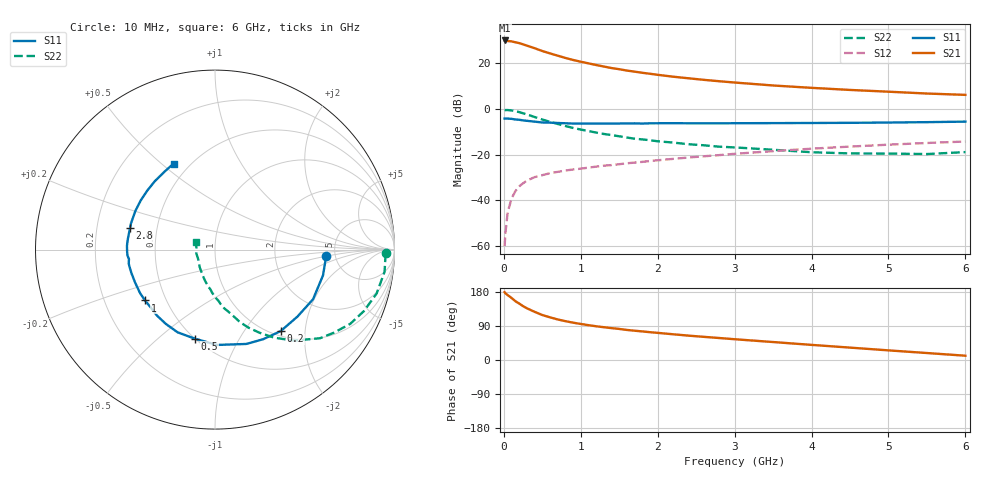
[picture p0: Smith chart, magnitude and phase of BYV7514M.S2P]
! SIEMENS Small Signal Semiconductors
! BFY420
! Si NPN RF SIEGET Grounded Emitter Transistor in MICRO-X
! VCE = 0.75 V  IC = 14 mA
! Common Emitter S-Parameters:  October  1996
# GHz  S  MA  R  50
!  f  S11  S21  S12  S22
! GHz  MAG  ANG  MAG  ANG  MAG  ANG  MAG  ANG
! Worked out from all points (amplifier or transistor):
!   36 points, 10 MHz to 6 GHz, reference 50 ohm
!   highest |S21| = 30.0 dB at 10 MHz (marker M1)
!   |S21| within 3 dB of that: start of sweep to 365.3 MHz
!   unconditionally stable (mu >= 1): 2.029 GHz to end of sweep
!   at 250 MHz: K = 0.25, MSG = 30.4 dB, |S12| = -32.5 dB
!   at 1.4 GHz: K = 0.87, MSG = 21.2 dB, |S12| = -24.5 dB
!   at 6 GHz: K = 1.11, MAG = 8.2 dB, |S12| = -14.2 dB
!   S11 on the Smith chart (normalised r, x): 10 MHz: 4.19, -0.50; 200 MHz: 1.09, -1.49; 500 MHz: 0.50, -0.67; 1 GHz: 0.38, -0.28; 2.8 GHz: 0.35, +0.11; 6 GHz: 0.41, +0.55
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0.01  0.6189 -3.4  31.77 179.0  0.001 98.9  0.9541 -1.3
0.02  0.6183 -5.6  31.72 176.0  0.0019 82.2  0.9503 -2.7
0.1  0.6124 -26.8  30.31 163.8  0.011 79.7  0.9332 -15.2
0.15  0.592 -39.0  28.97 155.2  0.016 73.3  0.8978 -22.4
0.2  0.5833 -51.1  27.76 148.9  0.0203 69.6  0.8593 -28.8
0.25  0.5669 -61.7  26.1 142.1  0.0238 64.5  0.8085 -34.9
0.3  0.554 -71.6  24.49 136.4  0.0272 61.7  0.7653 -40.2
0.4  0.5313 -88.8  21.49 127.1  0.0324 56.6  0.671 -49.1
0.5  0.5088 -102.8  18.64 118.7  0.0358 52.9  0.5912 -56.1
0.6  0.5058 -114.3  16.54 112.6  0.0396 50.9  0.5258 -61.8
0.7  0.4963 -123.5  14.76 107.0  0.0423 49.6  0.4731 -66.8
0.8  0.4896 -131.3  13.16 102.5  0.0452 47.8  0.4261 -71.1
1  0.4818 -144.0  10.87 95.1  0.0497 47.6  0.3565 -77.5
1.1  0.4829 -149.7  10.02 91.9  0.0524 48.1  0.3307 -81.1
1.4  0.4818 -161.3  7.911 84.1  0.0595 47.9  0.2702 -88.8
1.6  0.4854 -168.0  6.967 79.3  0.0651 47.8  0.2386 -94.1
2.2  0.491 177.5  5.117 67.9  0.0814 46.7  0.1851 -106.8
2.8  0.4883 165.8  4.071 58.0  0.0984 44.4  0.1504 -118.9
3.5  0.4932 154.2  3.285 47.4  0.1201 40.4  0.1288 -131.9
4.5  0.5004 138.9  2.625 32.7  0.1511 32.4  0.1071 -152.3
5.5  0.5177 122.7  2.19 18.4  0.1813 23.0  0.1038 174.2
6  0.5317 115.7  2.046 11.3  0.1951 18.0  0.1146 158.5
